PROGRAM Mannual
VAR
	//////////////////////手动////////////////////////////////////////////
	//输入
	move_up: BOOL;                     //上行按钮
    move_down: BOOL;                   //下行按钮
END_VAR

IF move_down THEN  
   solenoid_valve_down:=TRUE;                                    //控制下行电磁阀吸合，气缸下行 
   solenoid_valve_up:=FALSE;                                                                                 
END_IF
IF limit_switch_down=TRUE THEN                                   //触发下限位，下行电磁阀松开
   solenoid_valve_down:=FALSE;  
END_IF

IF move_up THEN   
   solenoid_valve_up:=TRUE;                                      //控制上行电磁阀吸合，气缸上行  
   solenoid_valve_down:=FALSE;                                                                                        
END_IF

IF limit_switch_up=TRUE THEN                                     //触发上限位，上行电磁阀松开
   solenoid_valve_up:=FALSE; 
END_IF

END_PROGRAM
